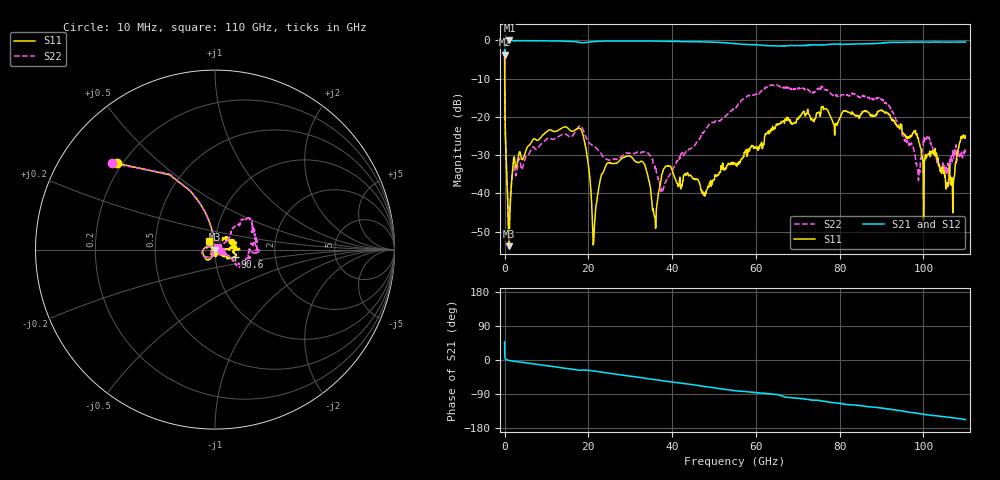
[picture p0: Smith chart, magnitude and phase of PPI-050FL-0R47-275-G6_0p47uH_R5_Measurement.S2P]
! Data measured by Modelithics Inc.  support@modelithics.com  813-866-6335  Tampa FL USA June 2025
! PPI-050FL-0R47-275-G6_0p47uH measured on 5-mil thick RO3003G2 board, mounted in 2-port shunt configuration on a 50-ohm transmission line
# GHz S RI R 50.0
!freq ReS11 ImS11 ReS21 ImS21 ReS12 ImS12 ReS22 ImS22
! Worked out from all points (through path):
!   1207 points, 10 MHz to 110 GHz, reference 50 ohm
!   highest |S21| = -0.01 dB at 1.174 GHz (marker M1); lowest = -3.7 dB at 10 MHz (marker M2)
!   group delay of S21, straight-line fit = 3.98 ps
!   lowest |S11| = -53.8 dB at 1.077 GHz (marker M3), VSWR 1.00, Z = 49.8 - j0.11 ohm
!   |S11| at or under -10 dB: 34.51 MHz to end of sweep
!   |S22| runs from -51.2 to -2.5 dB; largest |S21 - S12| = 0.081
!   S11 on the Smith chart (normalised r, x): 10 MHz: 0.18, +0.37; 90.6 GHz: 1.24, -0.11; 110 GHz: 0.93, +0.09
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0.01  -0.5483 0.4812  0.4395 0.4815  0.4395 0.4814  -0.5734 0.4802
0.2  -0.00629 0.0573  0.9936 0.0537  0.9935 0.0537  -0.00666 0.0575
1.07671  -0.00173 -0.0011  0.9981 -0.02  0.998 -0.0198  -0.00261 -0.000845
1.173799  -0.00179 -0.00325  0.998 -0.0239  0.9979 -0.0236  -0.00286 -0.00298
2.338865  -0.019 -0.0232  0.9811 -0.0623  0.9811 -0.062  -0.0206 -0.0151
6.70786  -0.0217 -0.0449  0.972 -0.1726  0.9718 -0.1729  -0.018 -0.036
18.35852  -0.0665 -0.0036  0.8324 -0.4184  0.8325 -0.4185  -0.0731 -0.0156
21.36827  0.00291 -0.00118  0.8445 -0.4706  0.8453 -0.4693  -0.0385 0.0156
23.79549  0.0142 -0.0149  0.8232 -0.5342  0.8243 -0.5326  -0.0252 0.0147
28.74702  0.00304 -0.0299  0.747 -0.6433  0.7474 -0.6429  -0.0312 0.0114
35.73741  -0.00169 -0.00479  0.6121 -0.7664  0.6064 -0.7712  0.00787 0.0213
36.7083  -0.00915 -0.00416  0.5899 -0.7821  0.5871 -0.7843  0.00917 0.0119
38.74716  -0.0181 -0.014  0.54 -0.812  0.5442 -0.8093  -0.00267 0.015
47.67933  -0.00211 0.00982  0.3314 -0.8968  0.3341 -0.8958  0.0527 0.0372
55.05808  0.0198 0.0142  0.1396 -0.8979  0.1468 -0.8968  0.0894 0.0961
73.4  0.08 0.0441  -0.2421 -0.8366  -0.1817 -0.8488  0.2032 0.0332
90.6  0.1097 -0.0421  -0.5728 -0.7337  -0.563 -0.7542  0.1348 -0.0789
91.7  0.0986 -0.0461  -0.59 -0.7304  -0.5968 -0.7346  0.1169 -0.0829
98.6  0.0427 -0.0314  -0.7356 -0.5998  -0.7301 -0.6096  0.0196 0.00719
100.7  0.00363 -0.029  -0.7686 -0.5558  -0.7602 -0.5709  0.0254 0.045
106.4  -0.00985 -0.0134  -0.8311 -0.4591  -0.8392 -0.4403  0.0217 -0.00802
110  -0.0326 0.0464  -0.8769 -0.3683  -0.885 -0.3607  0.0337 -0.0063
